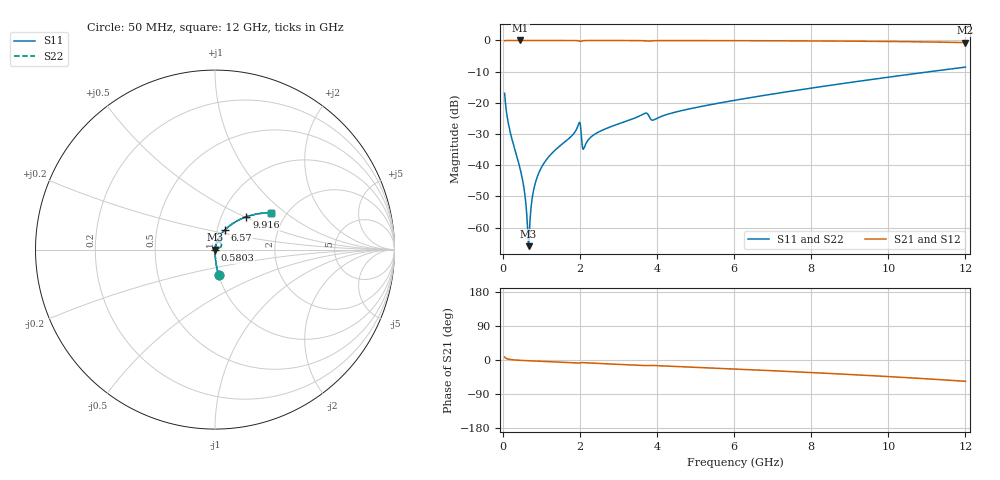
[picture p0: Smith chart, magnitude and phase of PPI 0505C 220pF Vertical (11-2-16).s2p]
# GHz S MA R 50
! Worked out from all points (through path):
!   1601 points, 50 MHz to 12 GHz, reference 50 ohm
!   highest |S21| = 0.00 dB at 460.8 MHz (marker M1); lowest = -0.7 dB at 12 GHz (marker M2)
!   group delay of S21, straight-line fit = 12.8 ps
!   lowest |S11| = -66.0 dB at 669.9 MHz (marker M3), VSWR 1.00, Z = 50.1 - j0.00313 ohm
!   |S11| at or under -10 dB: start of sweep to 11.08 GHz
!   |S22| runs from -66.0 to -8.6 dB; largest |S21 - S12| = 0
!   S11 on the Smith chart (normalised r, x): 50 MHz: 1.00, -0.29; 580.3 MHz: 1.00, -0.01; 6.57 GHz: 1.09, +0.25; 9.916 GHz: 1.31, +0.51; 12 GHz: 1.67, +0.80
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0.05  0.1422 -81.9  0.9896 8.0  0.9896 8.0  0.1422 -81.9
0.1919063  0.03456 -88.1  0.9991 1.4  0.9991 1.4  0.03456 -88.1
0.4607812  0.008315 -87.9  0.9995 -0.9  0.9995 -0.9  0.008315 -87.9
0.5802812  0.003177 -82.9  0.9995 -1.5  0.9995 -1.5  0.003177 -82.9
0.6325625  0.001353 -70.5  0.9995 -1.8  0.9995 -1.8  0.001353 -70.5
0.6699063  0.0005025 -3.6  0.9995 -2.0  0.9995 -2.0  0.0005025 -3.6
0.70725  0.001276 64.1  0.9994 -2.2  0.9994 -2.2  0.001276 64.1
0.7744688  0.003206 78.0  0.9994 -2.5  0.9994 -2.5  0.003206 78.0
0.8342188  0.004853 80.8  0.9994 -2.7  0.9994 -2.7  0.004853 80.8
1.043344  0.01011 82.9  0.9993 -3.7  0.9993 -3.7  0.01011 82.9
1.962  0.0443 66.5  0.9873 -8.2  0.9873 -8.2  0.0443 66.5
2.044156  0.02759 23.4  0.9759 -6.8  0.9759 -6.8  0.02759 23.4
2.118844  0.01945 65.1  0.9938 -7.3  0.9938 -7.3  0.01945 65.1
2.469875  0.03357 78.6  0.998 -9.2  0.998 -9.2  0.03357 78.6
3.664875  0.06684 68.3  0.9893 -14.6  0.9893 -14.6  0.06684 68.3
4.038312  0.05776 70.7  0.9939 -15.1  0.9939 -15.1  0.05776 70.7
6.025  0.11 65.3  0.992 -23.9  0.992 -23.9  0.11 65.3
6.570219  0.1253 62.9  0.9901 -26.3  0.9901 -26.3  0.1253 62.9
8.019156  0.1727 56.2  0.9826 -33.2  0.9826 -33.2  0.1727 56.2
9.916219  0.2534 46.2  0.9643 -43.2  0.9643 -43.2  0.2534 46.2
10.01331  0.2582 45.7  0.963 -43.8  0.963 -43.8  0.2582 45.7
12  0.3734 33.3  0.9237 -56.2  0.9237 -56.2  0.3734 33.3
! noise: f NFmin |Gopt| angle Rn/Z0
0.05  0.000325  0.8399  0.2732  0.0004299
1.372  0.003213  0.6109  3.916  0.00153
2.701  0.00578  0.5825  7.608  0.002512
4.031  0.01331  0.7088  11.62  0.008906
5.36  0.00939  0.5154  14.45  0.003333
6.682  0.01101  0.4949  17.53  0.003674
8.012  0.01298  0.4915  20.57  0.004261
9.341  0.01525  0.4978  23.54  0.005042
10.67  0.01789  0.5121  26.48  0.006082
12  0.02105  0.5336  29.43  0.007502
